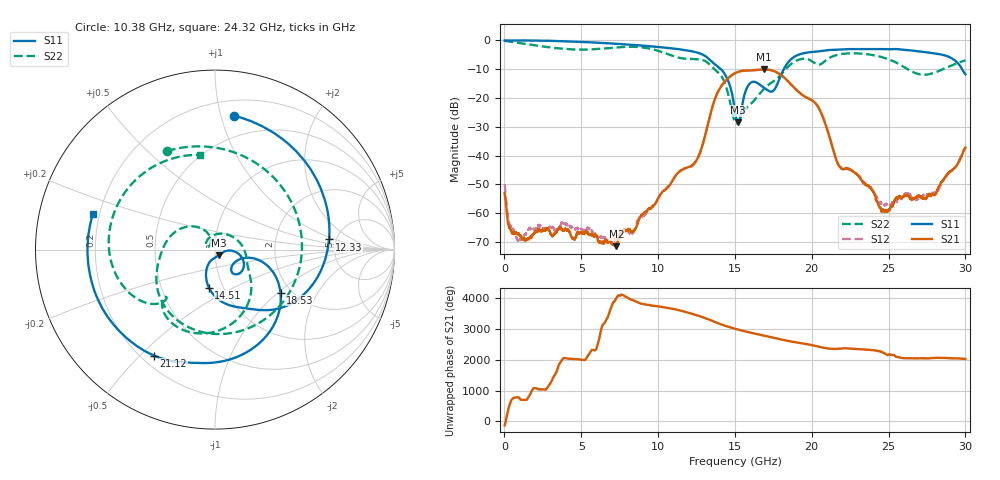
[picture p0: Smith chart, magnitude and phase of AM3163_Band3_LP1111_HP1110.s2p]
!Agilent Technologies,E8364B,MY43040894,A.07.50.67
!Agilent E8364B: A.07.50.67
!Date: Thursday, August 20, 2020 12:17:14
!Correction: S11(Full 2 Port(1,2))
!S21(Full 2 Port(1,2))
!S12(Full 2 Port(1,2))
!S22(Full 2 Port(1,2))
!S2P File: Measurements: S11, S21, S12, S22:
# Hz S  dB  R 50
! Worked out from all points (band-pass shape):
!   3201 points, 10 MHz to 30 GHz, reference 50 ohm
!   highest |S21| = -10.07 dB at 16.88 GHz (marker M1); lowest = -71.4 dB at 7.292 GHz (marker M2)
!   |S21| within 3 dB of the highest: 14.57 GHz to 18.24 GHz (3.673 GHz wide, 22.4 % of centre)
!   lowest |S11| = -28.4 dB at 15.2 GHz (marker M3), VSWR 1.08, Z = 51.9 - j3.38 ohm
!   |S11| at or under -10 dB: 14.1 GHz to 18.18 GHz (4.079 GHz wide, 25.3 % of centre); 29.79 GHz to end of sweep
!   |S22| runs from -28.8 to -0.1 dB; largest |S21 - S12| = 0.0054
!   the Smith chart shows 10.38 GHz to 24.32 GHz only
!   S11 on the Smith chart (normalised r, x): 10.38 GHz: 0.32, +1.10; 12.33 GHz: 4.35, +0.83; 14.51 GHz: 0.86, -0.38; 18.53 GHz: 1.76, -1.04; 21.12 GHz: 0.25, -0.55; 24.32 GHz: 0.17, +0.14
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1e7  -0.00 -2.0  -52.95 -132.2  -49.89 -130.8  -0.11 -5.0
1.256459e9  -0.01 -33.3  -68.48 -19.6  -67.98 -38.0  -1.12 -82.2
2.671612e9  -0.09 -70.6  -65.92 -52.9  -65.83 -46.9  -2.21 -162.1
5.014581e9  -0.51 -130.0  -67.02 -160.8  -65.64 -141.3  -3.20 75.8
7.291947e9  -1.16 172.5  -71.44 57.6  -68.78 23.2  -2.42 -48.9
8.454059e9  -1.58 141.1  -65.89 -46.7  -65.93 -7.7  -2.22 -115.2
1.000979e10  -2.27 94.1  -54.73 138.9  -54.84 137.6  -3.61 143.9
1.037529e10  -2.46 81.8  -52.08 106.4  -52.22 107.8  -4.28 116.0
1.144369e10  -3.10 43.0  -45.26 1.6  -45.41 0.0  -6.11 23.2
1.233402e10  -3.91 5.1  -42.74 -120.6  -43.08 -119.6  -6.43 -58.1
1.331806e10  -6.46 -44.2  -27.45 68.6  -27.54 70.9  -8.15 -144.7
1.450829e10  -13.39 -99.2  -13.38 -155.9  -13.21 -155.4  -17.58 120.8
1.5005e10  -24.72 -106.5  -11.38 130.4  -11.32 130.6  -28.29 130.7
1.520181e10  -28.38 -58.5  -10.92 103.2  -10.88 103.5  -28.46 152.4
1.687938e10  -16.39 -52.9  -10.07 -90.5  -9.98 -90.7  -16.85 15.5
1.852882e10  -7.20 -33.3  -14.58 87.7  -14.59 88.1  -8.78 -61.2
2.000958e10  -4.01 -91.3  -20.82 -41.0  -20.67 -40.3  -7.20 -132.2
2.111546e10  -3.33 -120.0  -32.83 -153.4  -32.68 -153.6  -6.16 -143.5
2.432064e10  -2.99 163.7  -56.93 125.6  -56.17 153.9  -5.45 99.1
2.500479e10  -3.04 146.6  -58.79 13.6  -57.18 29.2  -6.55 68.2
2.740399e10  -4.08 78.9  -55.02 -111.8  -53.75 -105.2  -11.90 -88.5
3e10  -11.74 -27.1  -37.24 -129.2  -37.06 -124.7  -6.95 130.8
